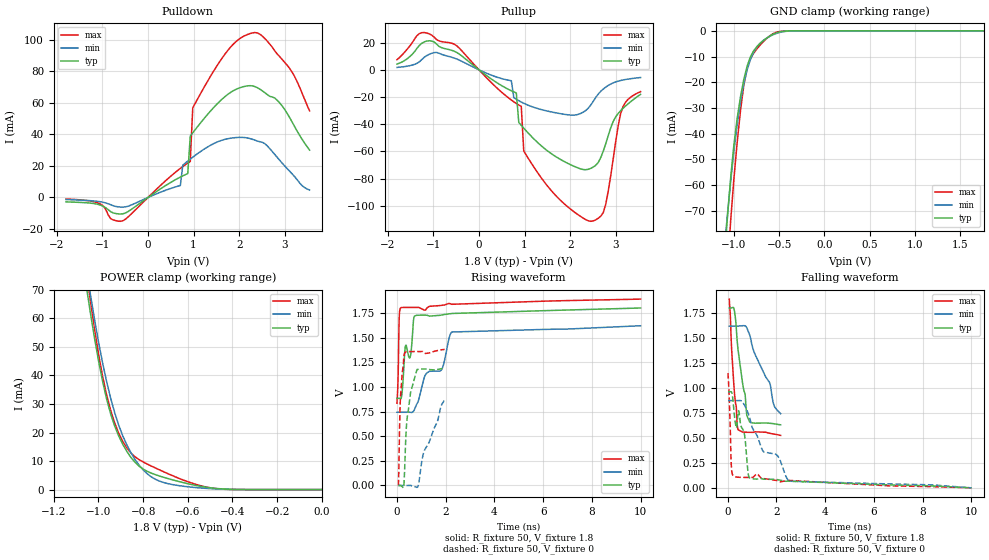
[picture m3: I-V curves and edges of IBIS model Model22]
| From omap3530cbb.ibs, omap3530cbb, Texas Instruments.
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| Model based on original model for OQ0163CS_7LM
|   Sub model OQ0163CS_7LM_DS0_1
[model]   Model22
|[Input Load]
|[Output Drive] FAST
|Voltage   1.8V
|Mode   3-STATE
Model_type   3-state
Polarity   Non-Inverting
Enable   Active-Low
Cref =  15.0000pF
Rref =  100.0000M
Vref =  0V
Vmeas =  0.9
C_comp   1.471p   1.219p   1.654p
[Temperature Range]   25   125   -40
[Voltage Range]   1.8   1.62   1.89
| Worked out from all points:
|   slope of the pulldown table from 0 to 0.27 V, typ, clamps not added: 50.1 ohm
|   slope of the pullup table from 0 to 0.27 V, typ, clamps not added: 40.2 ohm
|   GND clamp passes 1 mA (typ) near -0.54 V on its own axis
|   POWER clamp passes 1 mA (typ) near -0.53 V on its own axis
|   rising waveform, R_fixture 50, V_fixture 1.8: 20-80 % time 411ps typ, 1.15ns min, 49.5ps max; typ from 0.883 V to 1.8 V
|   rising waveform, R_fixture 50, V_fixture 0: 20-80 % time 242ps typ, 733ps min, 120ps max; typ from 0 V to 1.19 V
|   falling waveform, R_fixture 50, V_fixture 1.8: 20-80 % time 376ps typ, 836ps min, 231ps max; typ from 1.8 V to 0.631 V
|   falling waveform, R_fixture 50, V_fixture 0: 20-80 % time 363ps typ, 1.39ns min, 87.4ps max; typ from 0.963 V to 0 V
[POWER_clamp]
-1.8V     586.6mA    600.4mA    641.5mA
-1.055V   71.31mA    77.72mA    76.65mA
-1.036V   62.02mA    68.51mA    66.23mA
-1V       45.25mA    51.81mA    47.6mA
-981.8mV  38.06mA    44.48mA    39.84mA
-963.6mV  31.78mA    37.88mA    33.26mA
-927.3mV  22.24mA    26.91mA    23.34mA
-872.7mV  13.36mA    15.61mA    14.55mA
-781.8mV  6.402mA    5.553mA    8.957mA
-690.9mV  3.917mA    2.129mA    5.654mA
-490.9mV  560.2uA    303.2uA    525.6uA
0V        1.021nA    6.85nA     484.5pA
[Pulldown]
-1.8V     -2.794mA   -1.321mA   -1.013mA
-490.9mV  -9.78mA    -5.926mA   -13.68mA
709.1mV   12.91mA    7.574mA    18.43mA
763.6mV   13.7mA     20.47mA    19.62mA
872.7mV   15.15mA    23.06mA    21.83mA
927.3mV   38.86mA    24.31mA    22.83mA
981.8mV   40.94mA    25.53mA    56.76mA
1.691V    63.95mA    36.85mA    90.93mA
2.182V    70.72mA    37.7mA     103.3mA
2.455V    68.62mA    35.28mA    103.5mA
3.055V    53.27mA    18.28mA    83.74mA
3.545V    30mA       4.691mA    54.91mA
[Pullup]
-1.8V     4.285mA    1.799mA    7.469mA
-1.255V   19.54mA    7.627mA    27.35mA
-490.9mV  12.81mA    7.987mA    17.71mA
709.1mV   -15.4mA    -8.007mA   -22.19mA
818.2mV   -16.98mA   -21.6mA    -24.72mA
872.7mV   -38.66mA   -22.67mA   -25.85mA
927.3mV   -40.79mA   -23.66mA   -26.89mA
981.8mV   -42.88mA   -24.58mA   -59.72mA
2.455V    -72.41mA   -25.78mA   -111.4mA
2.782V    -54.23mA   -12.68mA   -98.79mA
3.164V    -28.18mA   -7.43mA    -26.77mA
3.545V    -18.02mA   -5.657mA   -16.05mA
[GND_clamp]
-1.8V     -511.9mA   -404mA     -763.6mA
-1.109V   -90.66mA   -85.99mA   -119mA
-1.073V   -73.05mA   -71.96mA   -94.34mA
-1.036V   -57.45mA   -58.82mA   -74.12mA
-1V       -44.37mA   -46.83mA   -57.58mA
-927.3mV  -25.68mA   -27.61mA   -31.09mA
-890.9mV  -18.99mA   -20.64mA   -21.3mA
-854.5mV  -13.83mA   -15.29mA   -14.76mA
-745.5mV  -6.156mA   -6.246mA   -7.023mA
-563.6mV  -1.279mA   -1.488mA   -1.068mA
-345.5mV  -12uA      -40.39uA   -6.042uA
1.764V    914.5pA    178nA      451pA
[Ramp]
dV/dt_f 0.73095974/0.38379942n 0.55947708/0.85717248n 0.83404804/0.23511458n
dV/dt_r 0.75622532/0.26487678n 0.57083634/0.77084163n  0.8583294/0.12546927n
R_load = 50
[Rising Waveform]
R_fixture = 50
V_fixture = 1.8
V_fixture_min = 1.62
V_fixture_max = 1.89
0s        883.3mV    742.6mV    834.2mV
94ps      883.6mV    742.6mV    1.719V
167.3ps   882.9mV    742.6mV    1.804V
339.2ps   1.405V     742.6mV    1.806V
541.7ps   1.303V     742.4mV    1.806V
797.2ps   1.726V     818.8mV    1.806V
1.176ns   1.728V     1.126V     1.78V
1.849ns   1.73V      1.183V     1.828V
2.253ns   1.744V     1.557V     1.838V
10ns      1.8V       1.62V      1.89V
[Rising Waveform]
R_fixture = 50
V_fixture = 0
V_fixture_min = 0
V_fixture_max = 0
60.42ps   412.6nV    320.8nV    639.1nV
109.2ps   529.4uV    -575.8nV   637.6mV
137.7ps   847.9uV    -190.9nV   872.8mV
268.8ps   -20.92mV   -1.371uV   1.264V
310.7ps   143.9mV    -5.839uV   1.34V
369ps     522.1mV    -23.57uV   1.355V
420.7ps   692.8mV    -32.43uV   1.357V
819.9ps   1.176V     -19.44mV   1.358V
1.089ns   1.181V     326.9mV    1.351V
1.954ns   1.19V      874.1mV    1.38V
[Falling Waveform]
R_fixture = 50
V_fixture = 1.8
V_fixture_min = 1.62
V_fixture_max = 1.89
65.25ps   1.8V       1.62V      1.89V
163.3ps   1.802V     1.62V      1.375V
260.9ps   1.791V     1.62V      999.2mV
426.2ps   1.378V     1.62V      582.3mV
714.5ps   931.3mV    1.622V     557.3mV
781.9ps   726.5mV    1.603V     556.7mV
897.6ps   661.4mV    1.534V     556.2mV
1.734ns   646.5mV    1.044V     545.9mV
1.914ns   641.1mV    818.6mV    537.8mV
2.171ns   631.3mV    742.6mV    525.5mV
[Falling Waveform]
R_fixture = 50
V_fixture = 0
V_fixture_min = 0
V_fixture_max = 0
11.29ps   962.6mV    874.1mV    1.15V
149.4ps   962.1mV    874.2mV    214.5mV
287.4ps   691.7mV    874.1mV    113mV
359.8ps   599.2mV    874mV      108.6mV
459ps     766.6mV    874.3mV    106.1mV
897.4ps   99.46mV    707.1mV    104.7mV
1.441ns   88.36mV    370.3mV    87.7mV
2.051ns   81.81mV    320.1mV    72.31mV
2.541ns   66.34mV    66.55mV    74.2mV
10.01ns   412.6nV    320.8nV    639.1nV
